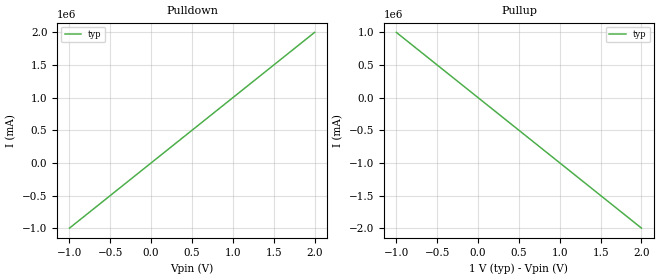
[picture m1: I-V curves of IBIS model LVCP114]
[IBIS Ver]   5.0
[File Name]  sn65lvcp114.ibs
[File Rev]   1.0
[Component]  LVCP114
[Manufacturer] Texas Instruments Incorporated
[Package]
R_pkg  0.0   NA   NA
L_pkg  0.0   NA   NA
C_pkg  0.0   NA   NA
[Pin]   signal_name   model_name   R_pin L_pin  C_pin
2p   IBIS_50ohm_Rx_2p   LVCP114
2n   IBIS_50ohm_Rx_2n   LVCP114
[Diff_Pin] inv_pin vdiff tdelay_typ tdelay_min tdelay_max
2p   2n   NA   NA   NA   NA
| Models and submodels in the file (1): LVCP114 (Input)
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[Model] LVCP114
Model_type Input
C_comp 0p 0p 0p
Vinl = 0.3
Vinh = 0.7
[Temperature_Range] 25 125 0
[Voltage Range] 1.0 1.0 1.0
[Algorithmic Model]
Executable Windows_VisualC++ExpressEdition9.0.30729_32 SN65LVCP114.dll SN65LVCP114.ami
|Executable Windows_VisualC++ExpressEdition9.0.30729_64 RX_model_x64.dll RX_model.ami
|Executable Linux_gcc4.6.1_64 RX_model_x64.so RX_model.ami
[End Algorithmic Model]
[Ramp]
|   typ   min   max
dV/dt_r   0.8/1.0ps   NA   NA
dV/dt_f   0.8/1.0ps   NA   NA
R_load = 0.001ohm
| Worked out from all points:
|   slope of the pulldown table from 0 to 0.15 V, typ, clamps not added: 1 mohm
|   slope of the pullup table from 0 to 0.15 V, typ, clamps not added: 1 mohm
[Pulldown]
|Voltage I(typ)   I(min)   I(max)
-1V       -1kA       NA         NA
0V        0A         NA         NA
2V        2kA        NA         NA
[Pullup]
-1V       1kA        NA         NA
0V        0A         NA         NA
2V        -2kA       NA         NA
[GND Clamp]
-6.6V     0A         0A         0A
0V        0A         0A         0A
6.6V      0A         0A         0A
[Power Clamp]
-6.6V     0A         0A         0A
0V        0A         0A         0A
6.6V      0A         0A         0A
